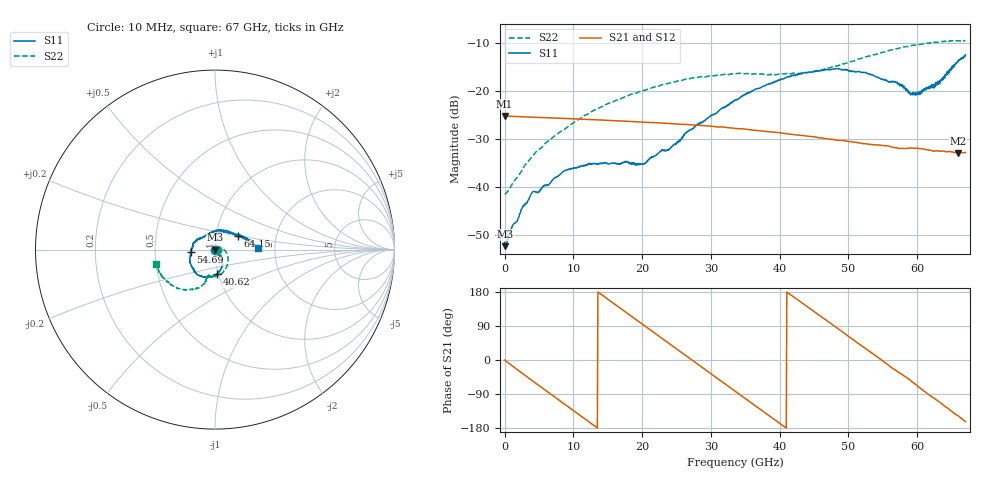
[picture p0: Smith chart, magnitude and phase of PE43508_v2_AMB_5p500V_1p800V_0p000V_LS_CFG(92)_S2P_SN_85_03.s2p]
!Keysight Technologies,N5227A,US51270237,A.10.43.00
!Date: Wednesday, August 22, 2018 17:16:15
!Correction: S11(Full 2 Port(1,3))
!S31(Full 2 Port(1,3))
!S13(Full 2 Port(1,3))
!S33(Full 2 Port(1,3))
!S2P File: Measurements: S11, S31, S13, S33:
# Hz S  dB  R 50
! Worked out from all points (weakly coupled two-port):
!   801 points, 10 MHz to 67 GHz, reference 50 ohm
!   highest |S21| = -25.13 dB at 10 MHz (marker M1); lowest = -32.9 dB at 65.91 GHz (marker M2)
!   lowest |S11| = -52.2 dB at 93.74 MHz (marker M3), VSWR 1.00, Z = 50.2 - j0.00816 ohm
!   |S11| at or under -10 dB: start of sweep to end of sweep
!   |S22| runs from -41.4 to -9.4 dB; largest |S21 - S12| = 0.00027
!   S11 on the Smith chart (normalised r, x): 10 MHz: 1.01, -0.00; 40.62 GHz: 0.98, -0.27; 54.69 GHz: 0.76, -0.02; 64.15 GHz: 1.27, +0.19; 67 GHz: 1.63, +0.03
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1e7  -51.45 -7.9  -25.13 -0.2  -25.14 -0.2  -41.28 -1.0
9.37375e7  -52.22 -1.9  -25.15 -1.4  -25.16 -1.4  -41.35 2.4
2.605862e9  -44.23 -42.4  -25.31 -35.5  -25.31 -35.5  -36.19 26.4
4.0294e9  -41.04 -54.0  -25.39 -54.5  -25.39 -54.5  -33.54 25.1
4.950512e9  -40.83 -60.4  -25.44 -66.7  -25.44 -66.7  -32.13 24.9
8.7187e9  -36.53 -84.5  -25.66 -116.6  -25.65 -116.6  -27.92 8.8
1.123082e10  -35.47 -89.8  -25.80 -149.7  -25.81 -149.7  -25.43 -4.4
2.002326e10  -35.09 -76.5  -26.40 94.6  -26.40 94.6  -19.91 -44.5
2.236791e10  -32.84 -64.6  -26.58 63.9  -26.58 63.8  -18.92 -54.6
2.395892e10  -32.04 -56.5  -26.72 43.0  -26.72 43.0  -18.30 -60.6
2.663852e10  -28.39 -52.3  -26.92 7.8  -26.92 7.8  -17.44 -70.5
3.3505e10  -21.91 -60.5  -27.71 -82.6  -27.71 -82.7  -16.35 -93.5
4.062269e10  -17.33 -85.5  -28.75 -175.3  -28.73 -175.3  -16.36 -105.2
4.472582e10  -15.98 -105.9  -29.42 131.3  -29.42 131.3  -16.00 -105.6
4.841028e10  -15.29 -125.6  -30.19 83.5  -30.17 83.4  -14.72 -106.3
5.469059e10  -17.46 -173.4  -31.23 1.5  -31.21 1.3  -12.01 -118.6
5.586291e10  -18.13 172.9  -31.40 -14.5  -31.39 -14.9  -11.52 -122.3
6.004979e10  -20.19 107.8  -31.84 -68.6  -31.84 -68.9  -10.38 -137.1
6.29806e10  -17.90 54.4  -32.38 -108.1  -32.41 -108.5  -9.82 -148.9
6.415292e10  -16.71 30.9  -32.56 -124.0  -32.63 -124.1  -9.62 -153.2
6.591141e10  -13.68 12.5  -32.86 -146.8  -32.91 -146.9  -9.49 -160.3
6.7e10  -12.40 2.0  -32.77 -162.4  -32.84 -162.4  -9.46 -166.2
